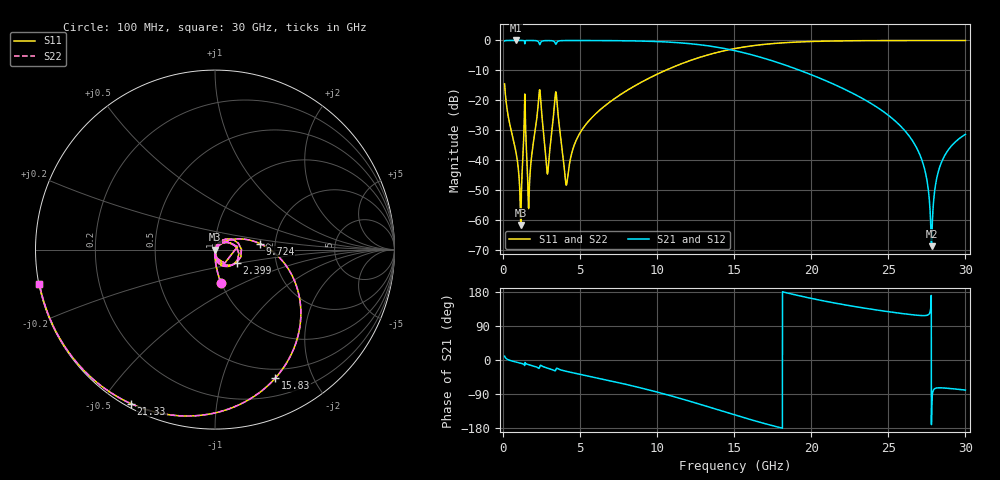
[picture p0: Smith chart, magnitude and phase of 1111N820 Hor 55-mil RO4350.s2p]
# GHz S MA R 50
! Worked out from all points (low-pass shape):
!   3201 points, 100 MHz to 30 GHz, reference 50 ohm
!   highest |S21| = -0.01 dB at 847.5 MHz (marker M1); lowest = -68.7 dB at 27.8 GHz (marker M2)
!   |S21| within 3 dB of the highest: start of sweep to 14.66 GHz
!   lowest |S11| = -61.6 dB at 1.147 GHz (marker M3), VSWR 1.00, Z = 50.1 - j0.00892 ohm
!   |S11| at or under -10 dB: start of sweep to 10.54 GHz
!   |S22| runs from -61.6 to 0.0 dB; largest |S21 - S12| = 1e-11
!   S11 on the Smith chart (normalised r, x): 100 MHz: 1.00, -0.38; 2.399 GHz: 1.26, -0.19; 9.724 GHz: 1.66, +0.12; 15.83 GHz: 0.39, -1.50; 21.33 GHz: 0.02, -0.59; 30 GHz: 0.00, -0.10
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0.1  0.1877 -79.9  0.982 10.1  0.982 10.1  0.1877 -79.9
0.8475  0.01313 -93.2  0.9993 -5.5  0.9993 -5.5  0.01313 -93.2
1.1465  0.0008291 -6.2  0.999 -8.5  0.999 -8.5  0.0008291 -6.2
1.380094  0.05271 56.0  0.9798 -13.0  0.9798 -13.0  0.05271 56.0
1.716469  0.00404 55.5  0.9983 -12.9  0.9983 -12.9  0.00404 55.5
2.398563  0.1408 -30.9  0.8632 -15.5  0.8632 -15.5  0.1408 -30.9
2.884438  0.005892 -11.7  0.9939 -21.2  0.9939 -21.2  0.005892 -11.7
3.46375  0.1206 -51.0  0.8924 -22.0  0.8924 -22.0  0.1206 -51.0
4.108469  0.003834 -19.5  0.9958 -29.9  0.9958 -29.9  0.003834 -19.5
5.089563  0.03123 47.2  0.9966 -38.5  0.9966 -38.5  0.03123 47.2
9.724063  0.2523 7.6  0.9637 -81.7  0.9637 -81.7  0.2523 7.6
10.06978  0.2784 4.0  0.9564 -85.4  0.9564 -85.4  0.2784 4.0
15.05  0.7324 -55.5  0.6738 -145.1  0.6738 -145.1  0.7324 -55.5
15.82553  0.791 -64.9  0.6041 -154.5  0.6041 -154.5  0.791 -64.9
20.03956  0.9605 -108.1  0.2648 162.2  0.2648 162.2  0.9605 -108.1
21.329  0.9779 -118.6  0.192 151.8  0.192 151.8  0.9779 -118.6
25.01978  0.9954 -143.3  0.05565 127.4  0.05565 127.4  0.9954 -143.3
27.02869  0.9969 -154.4  0.0126 117.5  0.0126 117.5  0.9969 -154.4
27.44916  0.997 -156.6  0.005507 117.5  0.005507 117.5  0.997 -156.6
27.80422  0.997 -158.4  0.0003653 -148.3  0.0003653 -148.3  0.997 -158.4
28.45828  0.9969 -161.6  0.009345 -73.5  0.009345 -73.5  0.9969 -161.6
30  0.9966 -168.9  0.02695 -79.3  0.02695 -79.3  0.9966 -168.9
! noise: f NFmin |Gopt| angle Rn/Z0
0.1  0.0006648  0.7343  1.268  0.0004995
3.417  0.09679  0.9316  24.99  0.3
6.743  0.01717  0.4497  46.31  0.004518
10.06  0.02456  0.4543  63.65  0.005735
13.39  0.03633  0.5259  79.32  0.008509
16.7  0.0578  0.6467  96.21  0.01462
20.03  0.1056  0.7857  115.3  0.03008
23.35  0.247  0.9025  134.7  0.08371
26.67  1.35  0.9811  152.7  0.922
30  0.977  0.9732  168.8  0.0814
